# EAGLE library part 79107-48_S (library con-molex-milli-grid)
RECEPTACAL
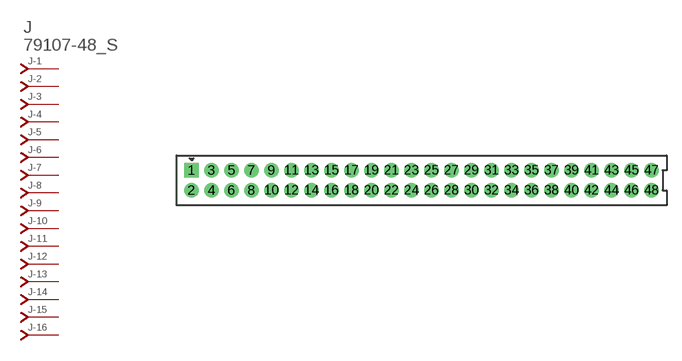
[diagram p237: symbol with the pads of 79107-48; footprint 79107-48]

Designator prefix J; gates -1=J-NV -2=J-N -3=J-N -4=J-N -5=J-N -6=J-N -7=J-N -8=J-N -9=J-N -10=J-N -11=J-N -12=J-N -13=J-N -14=J-N -15=J-N -16=J-N -17=J-N -18=J-N -19=J-N -20=J-N -21=J-N -22=J-N -23=J-N -24=J-N -25=J-N -26=J-N -27=J-N -28=J-N -29=J-N -30=J-N -31=J-N -32=J-N -33=J-N -34=J-N -35=J-N -36=J-N -37=J-N -38=J-N -39=J-N -40=J-N -41=J-N -42=J-N -43=J-N -44=J-N -45=J-N -46=J-N -47=J-N -48=J-N

## 79107-48_S  [79107-48]
1  -1:J  pas
2  -2:J  pas
3  -3:J  pas
4  -4:J  pas
5  -5:J  pas
6  -6:J  pas
7  -7:J  pas
8  -8:J  pas
9  -9:J  pas
10  -10:J  pas
11  -11:J  pas
12  -12:J  pas
13  -13:J  pas
14  -14:J  pas
15  -15:J  pas
16  -16:J  pas
17  -17:J  pas
18  -18:J  pas
19  -19:J  pas
20  -20:J  pas
21  -21:J  pas
22  -22:J  pas
23  -23:J  pas
24  -24:J  pas
25  -25:J  pas
26  -26:J  pas
27  -27:J  pas
28  -28:J  pas
29  -29:J  pas
30  -30:J  pas
31  -31:J  pas
32  -32:J  pas
33  -33:J  pas
34  -34:J  pas
35  -35:J  pas
36  -36:J  pas
37  -37:J  pas
38  -38:J  pas
39  -39:J  pas
40  -40:J  pas
41  -41:J  pas
42  -42:J  pas
43  -43:J  pas
44  -44:J  pas
45  -45:J  pas
46  -46:J  pas
47  -47:J  pas
48  -48:J  pas

## Footprint 79107-48 (pad centres in mm)
RECEPTACAL Dual Row, Vertical, Through-Hole
drill 0.914 square: 1 -23,1
drill 0.914: 2 -23,-1; 3 -21,1; 4 -21,-1; 5 -19,1; 6 -19,-1; 7 -17,1; 8 -17,-1; 9 -15,1; 10 -15,-1; 11 -13,1; 12 -13,-1; 13 -11,1; 14 -11,-1; 15 -9,1; 16 -9,-1; 17 -7,1; 18 -7,-1; 19 -5,1; 20 -5,-1; 21 -3,1; 22 -3,-1; 23 -1,1; 24 -1,-1; 25 1,1; 26 1,-1; 27 3,1; 28 3,-1; 29 5,1; 30 5,-1; 31 7,1; 32 7,-1; 33 9,1; 34 9,-1; 35 11,1; 36 11,-1; 37 13,1; 38 13,-1; 39 15,1; 40 15,-1; 41 17,1; 42 17,-1; 43 19,1; 44 19,-1; 45 21,1; 46 21,-1; 47 23,1; 48 23,-1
